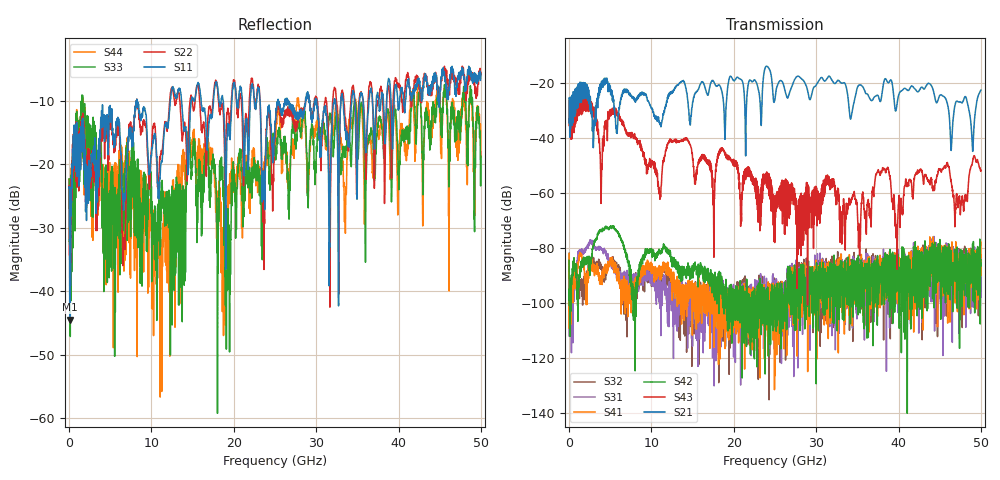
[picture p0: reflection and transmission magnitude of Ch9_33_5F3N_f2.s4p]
!Agilent Technologies,N5247A,US51170199,A.09.90.13
!Agilent N5247A: A.09.90.13
!Date: Wednesday, December 16, 2015 12:15:56
!Correction: S11(Full 4 Port(1,2,3,4))
!S12(Full 4 Port(1,2,3,4))
!S13(Full 4 Port(1,2,3,4))
!S14(Full 4 Port(1,2,3,4))
!S21(Full 4 Port(1,2,3,4))
!S22(Full 4 Port(1,2,3,4))
!S23(Full 4 Port(1,2,3,4))
!S24(Full 4 Port(1,2,3,4))
!S31(Full 4 Port(1,2,3,4))
!S32(Full 4 Port(1,2,3,4))
!S33(Full 4 Port(1,2,3,4))
!S34(Full 4 Port(1,2,3,4))
!S41(Full 4 Port(1,2,3,4))
!S42(Full 4 Port(1,2,3,4))
!S43(Full 4 Port(1,2,3,4))
!S44(Full 4 Port(1,2,3,4))
!S4P File: Measurements: <S11,S12,S13,S14>,
!<S21,S22,S23,S24>,
!<S31,S32,S33,S34>,
!<S41,S42,S43,S44>:
# Hz S  dB  R 50
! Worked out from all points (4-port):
!   3201 points, 10 MHz to 50 GHz, reference 50 ohm
!   strongest paths, dB at 10 MHz, 12.51 GHz, 25 GHz, 37.5 GHz, 50 GHz:
!     S21: -34.5, -23.5, -25.7, -24.4, -22.4
!     S43: -35.3, -41.5, -61.5, -52.0, -51.7
!     S42: -84.6, -84.4, -96.7, -92.8, -84.2
!     S41: -82.0, -88.8, -102.5, -100.7, -87.0
!     S31: -87.1, -94.8, -94.0, -102.0, -89.0
!     S32: -82.0, -95.5, -99.7, -96.8, -89.9
!   lowest |S11| = -44.5 dB at 88.11 MHz (marker M1), VSWR 1.01, Z = 50.4 + j0.48 ohm
!   |S11| at or under -10 dB: start of sweep to 8.214 GHz; 8.25 GHz to 12.28 GHz (4.032 GHz wide, 39.3 % of centre); 23.19 GHz to 25.35 GHz (2.159 GHz wide, 8.89 % of centre)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
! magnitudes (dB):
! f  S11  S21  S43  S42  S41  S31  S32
! 10 MHz  -23.7  -34.5  -35.3  -84.6  -82.0  -87.1  -82.0
! 88.11 MHz  -44.5  -39.6  -39.1  -101.6  -98.2  -100.1  -99.4
! 18.85 GHz  -13.1  -32.6  -45.0  -102.6  -102.7  -95.0  -101.7
! 35.22 GHz  -10.8  -20.6  -72.9  -86.4  -97.5  -85.0  -101.8
! 38.11 GHz  -8.9  -21.3  -51.0  -89.1  -97.5  -90.8  -94.3
! 39.75 GHz  -7.6  -29.0  -71.7  -92.2  -92.3  -85.4  -89.8
! 50 GHz  -5.7  -22.4  -51.7  -84.2  -87.0  -89.0  -89.9
